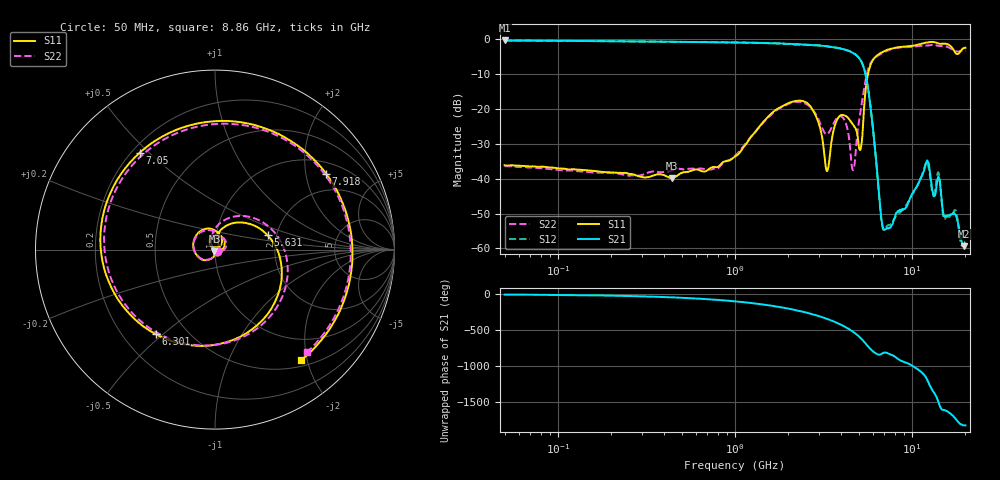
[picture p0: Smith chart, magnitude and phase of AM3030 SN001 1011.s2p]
# Hz S DB R 50
!freq MagS11 AngS11 MagS21 AngS21 MagS12 AngS12 MagS22 AngS22
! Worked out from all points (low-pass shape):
!   1601 points, 50 MHz to 20.05 GHz, reference 50 ohm
!   highest |S21| = -0.33 dB at 50 MHz (marker M1); lowest = -59.3 dB at 19.6 GHz (marker M2)
!   |S21| within 3 dB of the highest: start of sweep to 4.398 GHz
!   lowest |S11| = -39.8 dB at 439.1 MHz (marker M3), VSWR 1.02, Z = 49.7 - j0.97 ohm
!   |S11| at or under -10 dB: start of sweep to 5.648 GHz
!   |S22| runs from -39.2 to -1.6 dB; largest |S21 - S12| = 0.017
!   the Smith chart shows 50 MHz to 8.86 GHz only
!   S11 on the Smith chart (normalised r, x): 50 MHz: 1.02, -0.02; 5.631 GHz: 1.79, +0.32; 6.301 GHz: 0.34, -0.47; 7.05 GHz: 0.23, +0.47; 7.918 GHz: 1.36, +2.61; 8.86 GHz: 0.60, -1.90
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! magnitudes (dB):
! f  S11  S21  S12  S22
! 50 MHz  -36.2  -0.3  -0.4  -36.4
! 135.9 MHz  -37.5  -0.5  -0.5  -37.9
! 369.6 MHz  -38.7  -0.7  -0.7  -38.1
! 439.1 MHz  -39.8  -0.7  -0.7  -37.7
! 1.005 GHz  -33.6  -0.9  -0.9  -33.4
! 1.73 GHz  -20.0  -1.2  -1.1  -20.3
! 2.722 GHz  -19.9  -1.6  -1.7  -19.9
! 3.308 GHz  -37.8  -2.0  -2.0  -27.3
! 3.687 GHz  -24.4  -2.3  -2.3  -23.3
! 4.08 GHz  -21.7  -2.8  -2.8  -22.5
! 4.652 GHz  -24.5  -3.9  -3.9  -37.5
! 5.127 GHz  -31.5  -6.0  -6.0  -20.6
! 5.631 GHz  -10.3  -13.5  -13.5  -9.0
! 6.301 GHz  -4.8  -35.6  -35.9  -5.0
! 6.715 GHz  -3.8  -51.2  -51.8  -4.1
! 7.05 GHz  -3.3  -54.6  -54.5  -3.6
! 7.402 GHz  -2.9  -54.2  -53.3  -3.1
! 7.918 GHz  -2.5  -51.6  -51.7  -2.6
! 8.86 GHz  -2.1  -48.8  -48.9  -2.3
! 12.23 GHz  -0.9  -34.8  -35.3  -1.8
! 19.6 GHz  -2.5  -59.3  -58.9  -3.2
! 20.05 GHz  -2.4  -59.0  -58.0  -3.2
